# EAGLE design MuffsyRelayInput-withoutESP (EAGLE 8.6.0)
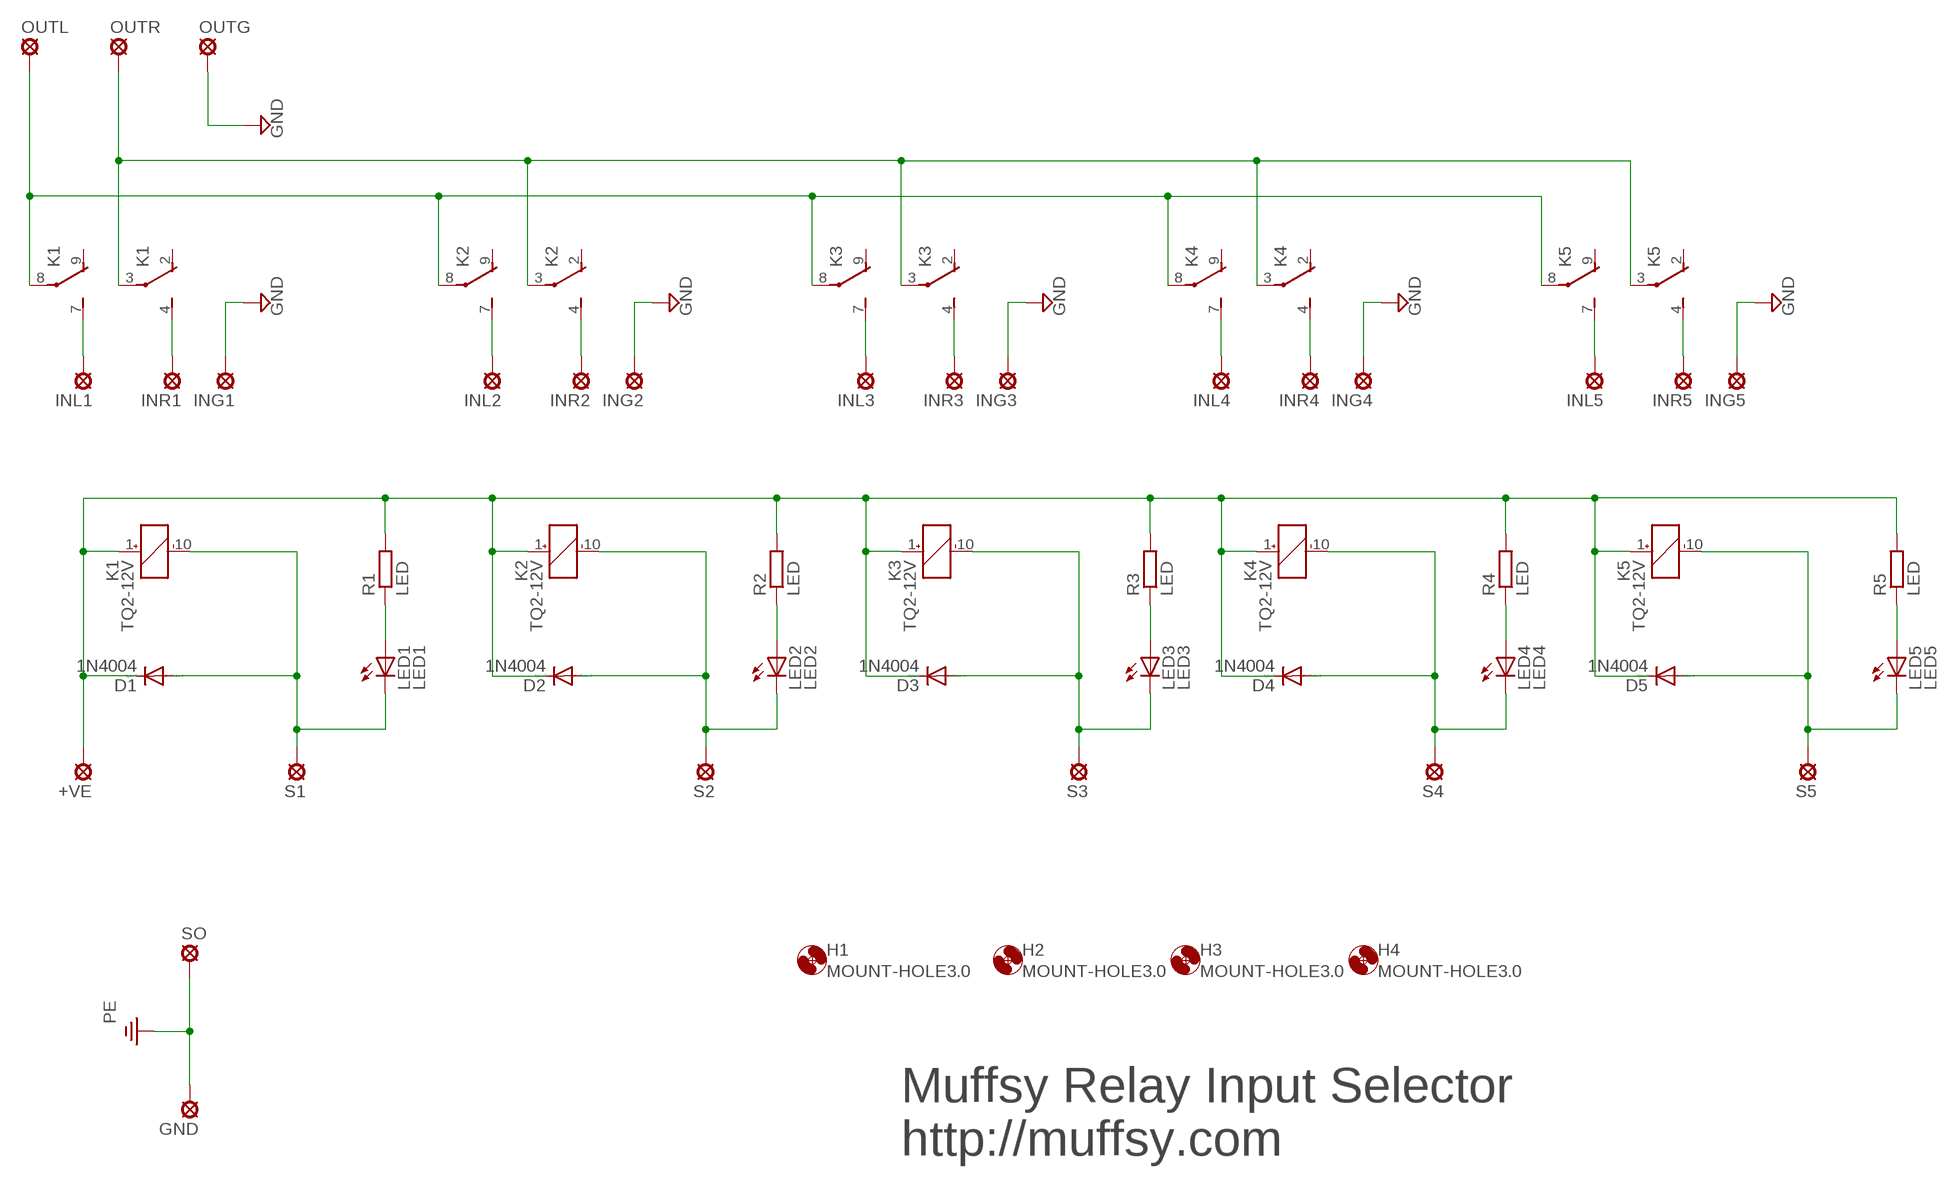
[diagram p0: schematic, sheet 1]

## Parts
+VE  SE11  [SE11]
D1  1N4004  [DO41-10]
D2  1N4004  [DO41-10]
D3  1N4004  [DO41-10]
D4  1N4004  [DO41-10]
D5  1N4004  [DO41-10]
GND  SE11  [SE11]
H1  MOUNT-HOLE3.0  [3,0]
H2  MOUNT-HOLE3.0  [3,0]
H3  MOUNT-HOLE3.0  [3,0]
H4  MOUNT-HOLE3.0  [3,0]
ING1  SE11  [SE11]
ING2  SE11  [SE11]
ING3  SE11  [SE11]
ING4  SE11  [SE11]
ING5  SE11  [SE11]
INL1  SE11  [SE11]
INL2  SE11  [SE11]
INL3  SE11  [SE11]
INL4  SE11  [SE11]
INL5  SE11  [SE11]
INR1  SE11  [SE11]
INR2  SE11  [SE11]
INR3  SE11  [SE11]
INR4  SE11  [SE11]
INR5  SE11  [SE11]
K1  TQ2-12V  [TQ2]
K2  TQ2-12V  [TQ2]
K3  TQ2-12V  [TQ2]
K4  TQ2-12V  [TQ2]
K5  TQ2-12V  [TQ2]
LED1  LED1  LED5MM  [LED5MM]
LED2  LED2  LED5MM  [LED5MM]
LED3  LED3  LED5MM  [LED5MM]
LED4  LED4  LED5MM  [LED5MM]
LED5  LED5  LED5MM  [LED5MM]
OUTG  SE11  [SE11]
OUTL  SE11  [SE11]
OUTR  SE11  [SE11]
R1  LED  R-EU_0207/10  [0207/10]
R2  LED  R-EU_0207/10  [0207/10]
R3  LED  R-EU_0207/10  [0207/10]
R4  LED  R-EU_0207/10  [0207/10]
R5  LED  R-EU_0207/10  [0207/10]
S1  SE11  [SE11]
S2  SE11  [SE11]
S3  SE11  [SE11]
S4  SE11  [SE11]
S5  SE11  [SE11]
SO  SE11  [SE11]

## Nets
GND: ING1.MP ING2.MP ING3.MP ING4.MP ING5.MP OUTG.MP
N$1: INL2.MP K2.7(2:S)
N$2: INL1.MP K1.7(2:S)
N$3: INR1.MP K1.4(1:S)
N$4: INR2.MP K2.4(1:S)
N$5: INL3.MP K3.7(2:S)
N$6: INR3.MP K3.4(1:S)
N$7: INL4.MP K4.7(2:S)
N$8: INR4.MP K4.4(1:S)
N$9: INL5.MP K5.7(2:S)
N$10: INR5.MP K5.4(1:S)
N$11: LED1.A R1.1
N$12: K1.3(1:P) K2.3(1:P) K3.3(1:P) K4.3(1:P) K5.3(1:P) OUTR.MP
N$13: K1.8(2:P) K2.8(2:P) K3.8(2:P) K4.8(2:P) K5.8(2:P) OUTL.MP
N$14: LED3.A R3.1
N$15: +VE.MP D1.C D2.C D3.C D4.C D5.C K1.1(_:+) K2.1(_:+) K3.1(_:+) K4.1(_:+) K5.1(_:+) R1.2 R2.2 R3.2 R4.2 R5.2
N$16: LED2.A R2.1
N$18: LED4.A R4.1
N$20: D1.A K1.10(_:-) LED1.K(C) S1.MP
N$21: D2.A K2.10(_:-) LED2.K(C) S2.MP
N$22: D3.A K3.10(_:-) LED3.K(C) S3.MP
N$23: D4.A K4.10(_:-) LED4.K(C) S4.MP
N$24: D5.A K5.10(_:-) LED5.K(C) S5.MP
N$26: LED5.A R5.1
PE: GND.MP SO.MP
Unconnected: K1.2(1:O) K1.9(2:O) K2.2(1:O) K2.9(2:O) K3.2(1:O) K3.9(2:O) K4.2(1:O) K4.9(2:O) K5.2(1:O) K5.9(2:O)

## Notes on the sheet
- Muffsy Relay Input Selector
- http://muffsy.com

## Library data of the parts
+VE GND ING1-ING5 INL1-INL5 INR1-INR5 OUTG OUTL OUTR S1-S5 SO = relswitch:SE11: SOLDER PAD
D1-D5 = relswitch:1N4004: DIODE
H1-H4 = relswitch:MOUNT-HOLE: MOUNTING HOLE with drill center marker
K1-K5 = relswitch:TQ2?*: LOW PROFILE 2 FORM C RELAY NAiS Source: http://www.mew-europe.com/.. en_ds_61020_0001.pdf Source: http://www.mew-europe.com/.. en_ds_61020_0004.pdf; MF: AROMAT/ MATSUSHITA; MPN: TQ2-12V; OC_FARNELL: 1200949; OC_NEWARK: 64K3197
LED1-LED5 = led:LED: LED
R1-R5 = rcl:R-EU_: RESISTOR, European symbol; SPICEPREFIX: R

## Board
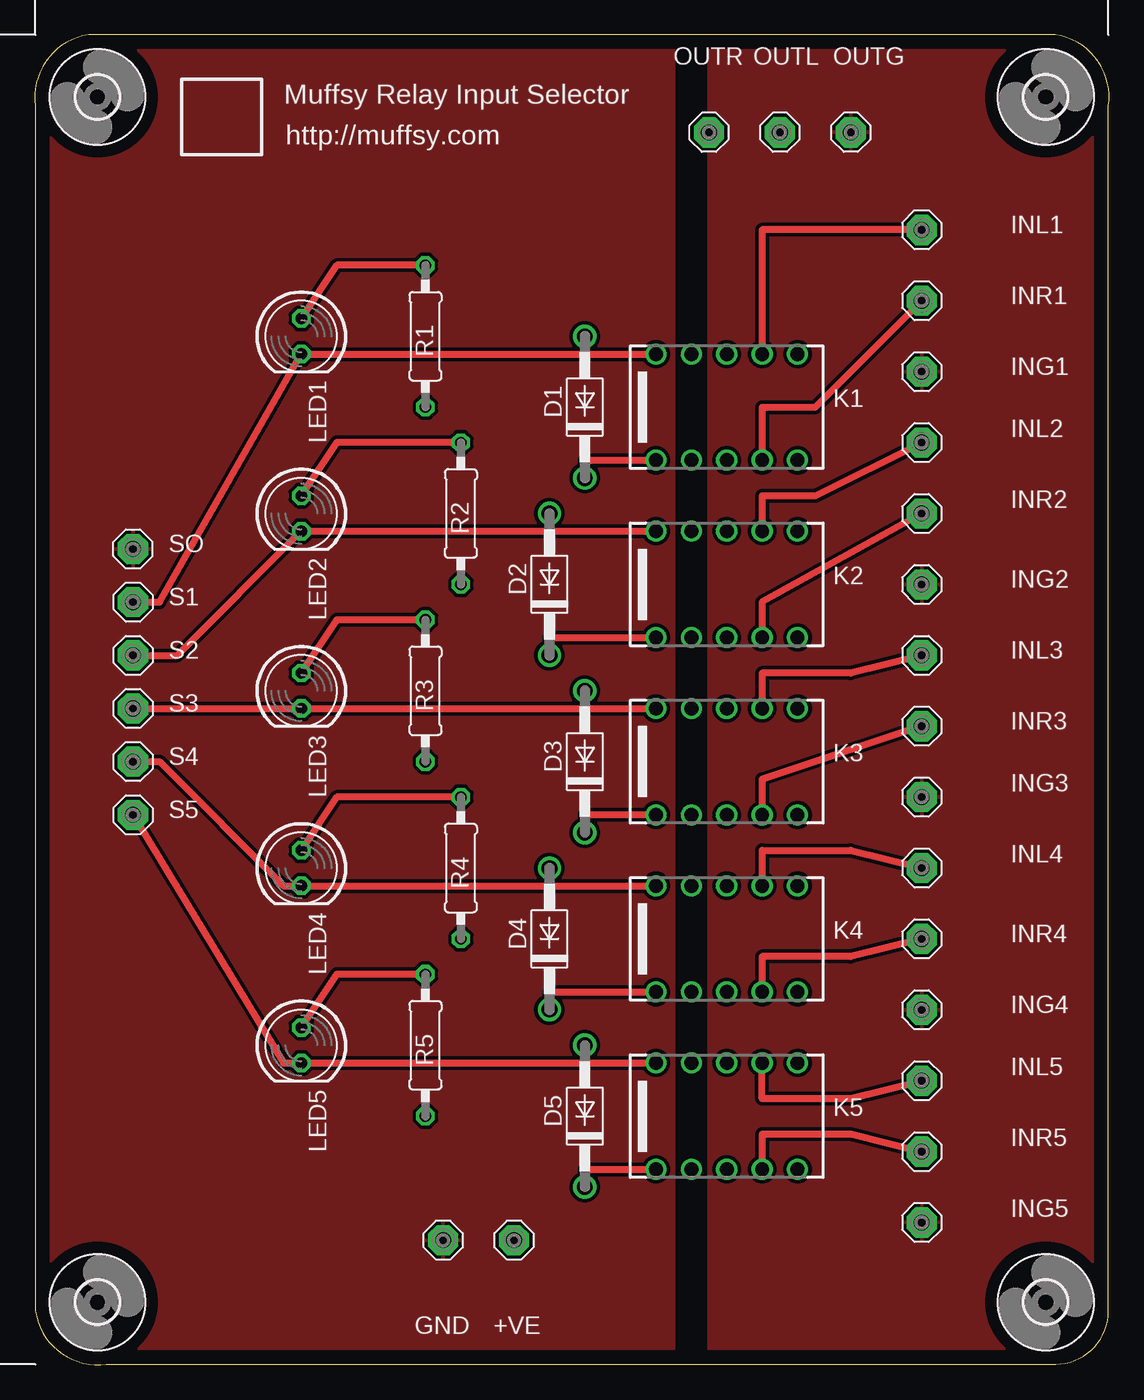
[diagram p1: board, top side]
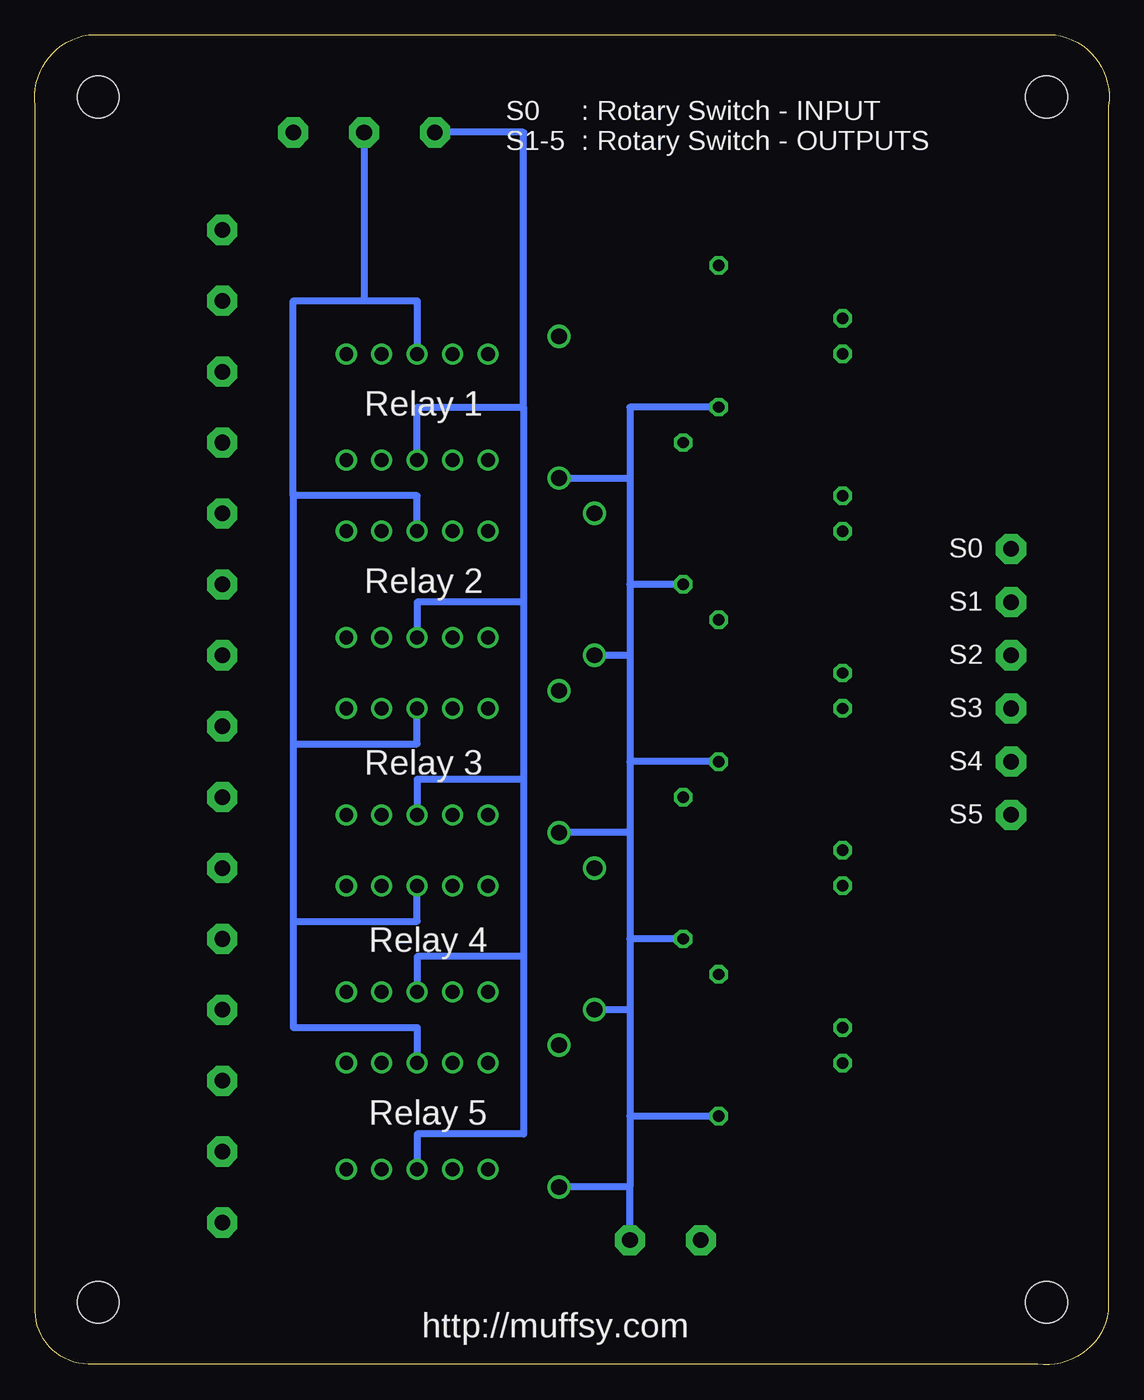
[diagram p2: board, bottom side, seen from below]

Size 76.97 x 95.27 mm. Coordinates in mm from the lower left corner, seen from the top.
Outline: 76.93,3.83 76.93,90.19 arc90 73.12,95.27 3.85,95.27 arc90 0.04,90.19 0.04,3.85 arc90 5.12,0.04 73.14,0.04 arc90 76.93,3.83
Copper layers (1*16): Top 0.035mm / dielectric 1.5mm / Bottom 0.035mm
Design rules "default": minimum track width 6mil, minimum drill 0.35mm, track to track 6mil, track to pad 6mil, pad to pad 6mil, via to via 6mil, smd to smd 6mil, copper to edge 40mil, drill to drill 6mil, minimum pad ring 10mil, minimum via ring 8mil, stop-mask expansion 4mil, vias tented up to drill 0mil, thermal gap 10mil

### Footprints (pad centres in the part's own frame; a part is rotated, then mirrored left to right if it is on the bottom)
SE11 = drill 1.118 pad 2.159 octagon: MP 0,0
DO41-10 = drill 1.118: A 5.08,0; C -5.08,0
3,0 = hole 3: 0,0
TQ2 = drill 1: 1 -5.08,-3.81; 2 -2.54,-3.81; 3 0,-3.81; 4 2.54,-3.81; 5 5.08,-3.81; 6 5.08,3.81; 7 2.54,3.81; 8 0,3.81; 9 -2.54,3.81; 10 -5.08,3.81
LED5MM = drill 0.813 octagon: A -1.27,0; K 1.27,0
0207/10 = drill 0.813 octagon: 1 -5.08,0; 2 5.08,0

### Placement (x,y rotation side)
+VE  34.33,8.91 270 top
D1  39.41,68.6 90 top
D2  36.87,55.9 90 top
D3  39.41,43.2 90 top
D4  36.87,30.5 90 top
D5  39.41,17.8 90 top
GND  29.25,8.91 270 top
H1  72.43,4.47 0 top
H2  4.49,4.47 0 top
H3  72.43,90.83 0 top
H4  4.49,90.83 0 top
ING1  63.54,71.14 0 top
ING2  63.54,55.9 0 top
ING3  63.54,40.66 0 top
ING4  63.54,25.42 0 top
ING5  63.54,10.18 0 top
INL1  63.54,81.3 0 top
INL2  63.54,66.06 0 top
INL3  63.54,50.82 0 top
INL4  63.54,35.58 0 top
INL5  63.54,20.34 0 top
INR1  63.54,76.22 0 top
INR2  63.54,60.98 0 top
INR3  63.54,45.74 0 top
INR4  63.54,30.5 0 top
INR5  63.54,15.26 0 top
K1  49.57,68.6 0 top
K2  49.57,55.9 0 top
K3  49.57,43.2 0 top
K4  49.57,30.5 0 top
K5  49.57,17.8 0 top
LED1  19.09,73.68 270 top
LED2  19.09,60.98 270 top
LED3  19.09,48.28 270 top
LED4  19.09,35.58 270 top
LED5  19.09,22.88 270 top
OUTG  58.46,88.29 270 top
OUTL  53.38,88.29 270 top
OUTR  48.3,88.29 270 top
R1  27.98,73.68 270 top
R2  30.52,60.98 270 top
R3  27.98,48.28 270 top
R4  30.52,35.58 270 top
R5  27.98,22.88 270 top
S1  7.03,54.63 0 top
S2  7.03,50.82 0 top
S3  7.03,47.01 0 top
S4  7.03,43.2 0 top
S5  7.03,39.39 0 top
SO  7.03,58.44 180 top

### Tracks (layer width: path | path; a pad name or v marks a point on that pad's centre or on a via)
GND
  pour Top (isolate 0.254): 76.88,0.02 76.88,95.27 48.3,95.27 48.3,0.02
N$1
  Top 0.508: K2.7 52.11,62.25 55.92,62.25 INL2.MP
N$2
  Top 0.508: INL1.MP 52.11,81.3 K1.7
N$3
  Top 0.508: K1.4 52.11,68.6 55.92,68.6 INR1.MP
N$4
  Top 0.508: INR2.MP 52.11,54.63 K2.4
N$5
  Top 0.508: INL3.MP 58.46,49.55 52.11,49.55 K3.7
N$6
  Top 0.508: INR3.MP 52.11,41.93 K3.4
N$7
  Top 0.508: K4.7 52.11,36.85 58.46,36.85 INL4.MP
N$8
  Top 0.508: INR4.MP 58.46,29.23 52.11,29.23 K4.4
N$9
  Top 0.508: K5.7 52.11,19.07 58.46,19.07 INL5.MP
N$10
  Top 0.508: K5.4 52.11,16.53 58.46,16.53 INR5.MP
N$11
  Top 0.508: R1.1 21.63,78.76 LED1.A
N$12
  Bottom 0.508: K1.3 49.57,68.6 41.95,68.6 | 41.95,68.6 41.95,54.63 | 41.95,54.63 49.57,54.63 K2.3 | 41.95,54.63 41.95,41.93 | 41.95,41.93 49.57,41.93 K3.3 | 41.95,41.93 41.95,29.23 | 41.95,29.23 49.57,29.23 K4.3 | 41.95,29.23 41.95,16.53 49.57,16.53 K5.3 | 41.95,68.6 41.95,88.29 OUTR.MP
N$13
  Bottom 0.508: 53.38,76.22 58.46,76.22 58.46,62.25 | 53.38,76.22 49.57,76.22 K1.8 | K2.8 49.57,62.25 58.46,62.25 | 58.46,62.25 58.46,44.47 | 58.46,44.47 49.57,44.47 K3.8 | 58.46,44.47 58.46,31.77 | 58.46,31.77 49.57,31.77 K4.8 | 58.46,31.77 58.46,24.15 49.57,24.15 K5.8 | OUTL.MP 53.38,76.22
N$14
  Top 0.508: R3.1 21.63,53.36 LED3.A
N$15
  Top 0.508: K1.1 39.41,64.79 D1.C | D2.C 36.87,52.09 K2.1 | D5.C 39.41,13.99 K5.1 | D4.C 36.87,26.69 K4.1 | K3.1 39.41,39.39 D3.C
  Bottom 0.508: 34.33,50.82 D2.C | 34.33,38.12 D3.C | 34.33,12.72 D5.C | 34.33,63.52 34.33,55.9 | 34.33,55.9 34.33,50.82 | 34.33,50.82 34.33,43.2 | 34.33,43.2 34.33,38.12 | 34.33,38.12 34.33,30.5 | 34.33,30.5 34.33,25.42 | 34.33,25.42 D4.C | 34.33,25.42 34.33,17.8 | 34.33,17.8 34.33,12.72 | D1.C 34.33,63.52 | +VE.MP 34.33,12.72 | R5.2 34.33,17.8 | R4.2 34.33,30.5 | R3.2 34.33,43.2 | R2.2 34.33,55.9 | R1.2 34.33,68.6 34.33,63.52
N$16
  Top 0.508: R2.1 21.63,66.06 LED2.A
N$18
  Top 0.508: R4.1 21.63,40.66 LED4.A
N$20
  Top 0.508: 39.41,72.41 K1.10 | 39.41,72.41 D1.A | S1.MP 8.93,54.63 LED1.K 39.41,72.41
N$21
  Top 0.508: D2.A 36.87,59.71 | 36.87,59.71 K2.10 | S2.MP 10.2,50.82 LED2.K 36.87,59.71
N$22
  Top 0.508: D3.A 39.41,47.01 | 39.41,47.01 K3.10 | S3.MP LED3.K 39.41,47.01
N$23
  Top 0.508: D4.A 36.87,34.31 | 36.87,34.31 K4.10 | S4.MP 8.93,43.2 17.82,34.31 LED4.K 36.87,34.31
N$24
  Top 0.508: D5.A 39.41,21.61 | 39.41,21.61 K5.10 | S5.MP 17.82,21.61 LED5.K 39.41,21.61
N$26
  Top 0.508: R5.1 21.63,27.96 LED5.A
PE
  pour Top (isolate 0.254, rank 5): 0.04,95.27 0.04,0.02 45.76,0.02 45.76,95.27

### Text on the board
tNames: Muffsy Relay Input Selector | http://muffsy.com
bNames: : Rotary Switch - INPUT / : Rotary Switch - OUTPUTS | S0 / S1-5 | Relay 1 | S0 | Relay 2 | S1 | S2 | S3 | S4 | Relay 3 | S5 | Relay 4 | Relay 5 | http://muffsy.com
